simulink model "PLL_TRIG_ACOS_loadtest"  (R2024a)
settings: Solver=VariableStepAuto  StartTime=0.0  StopTime=1  RelTol=1e-3
libraries: spsIGBTDiodeLib x6, spsThreePhaseSeriesRLCBranchLib x6, spsDiodeLib x6, spsGroundLib x4, spsThreePhaseBreakerLib x4, spsThreePhaseVIMeasurementLib x3, spsSeriesRLCBranchLib x3, spsMultimeterLib x3, spsThreePhaseSourceLib x2, spsTHDLib x2, spsPower3phInstantaneousLib x2, spsPVArrayLib x1

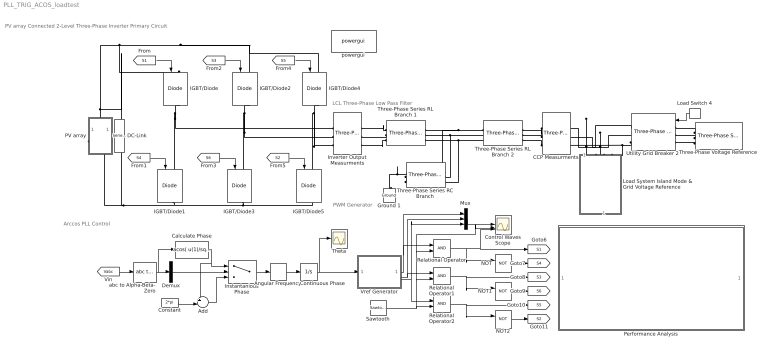
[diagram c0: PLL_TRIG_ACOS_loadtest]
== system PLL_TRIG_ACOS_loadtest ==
  note: PV array Connected 2-Level Three-Phase Inverter Primary Circuit
  note: LCL Three-Phase Low Pass Filter
  note: PWM Generator
  note: Arccos PLL Control
  Add : Sum  Inputs=+-|
  Angular Frequency : Derivative
  CCP Measurments : spsThreePhaseVIMeasurementLib/Three-Phase V-I Measurement  VoltageMeasurement=phase-to-phase  SetLabelV=on  LabelV=Vabc  Vpu=off  VpuLL=off  CurrentMeasurement=yes  SetLabelI=on  LabelI=Iabc  Ipu=off  Pbase=100e6  Vbase=500e3  OutputType=Complex  PhasorSimulation=off  PSBequivalent=0
  Calculate Phase : Fcn  Expr=acos( u(1)/sqrt( u(1)^2 + u(2)^2 ) )
  Constant : Constant  Value=2*pi
  Continuous Phase : Integrator
  Control Waves Scope : Scope  NumInputPorts=3
  DC-Link : spsSeriesRLCBranchLib/Series RLC Branch  LConnTagsString=__new0  RConnTagsString=__new0  BranchType=RC  Resistance=20e-3  Inductance=1e-3  SetiL0=off  InitialCurrent=0  Capacitance=81e-6  Setx0=off  InitialVoltage=0  Measurements=None
  Demux : Demux  Outputs=3
  Ground 1 : spsGroundLib/Ground  LConnTagsString=a
  IGBT/Diode{,1..5} (6 alike) : spsIGBTDiodeLib/IGBT//Diode  Ron=1e-3  Rs=1e5  Cs=inf  Measurements=off
  Instantanious Phase : Switch  Criteria=u2 > Threshold
  Inverter Output Measurments : spsThreePhaseVIMeasurementLib/Three-Phase V-I Measurement  VoltageMeasurement=phase-to-phase  SetLabelV=on  LabelV=Vinv  Vpu=off  VpuLL=off  CurrentMeasurement=yes  SetLabelI=on  LabelI=Iinv  Ipu=off  Pbase=100e6  Vbase=500e3  OutputType=Complex  PhasorSimulation=off  PSBequivalent=0
  Load Switch 4 : DiscretePulseGenerator  PulseType=Time based  Period=1.2  PulseWidth=50  PhaseDelay=0.6
  Load System Island Mode & Grid Voltage Reference : Subsystem
  Mux : Mux  Inputs=3
  NOT : Logic  Operator=NOT  IconShape=distinctive  AllPortsSameDT=off  OutDataTypeStr=boolean
  NOT1 : Logic  Operator=NOT  IconShape=distinctive  AllPortsSameDT=off  OutDataTypeStr=boolean
  NOT2 : Logic  Operator=NOT  IconShape=distinctive  AllPortsSameDT=off  OutDataTypeStr=boolean
  PV array : Subsystem
  Performance Analysis : Subsystem
  Relational Operator : RelationalOperator  OutDataTypeStr=boolean  RndMeth=Simplest
  Relational Operator1 : RelationalOperator  OutDataTypeStr=boolean  RndMeth=Simplest
  Relational Operator2 : RelationalOperator  OutDataTypeStr=boolean  RndMeth=Simplest
  Sawtooth : spsSawtoothGeneratorLib/Sawtooth Generator  Freq=1e4  Phase=0  Ts=0
  Theta : Scope
  Three-Phase Series RC Branch : spsThreePhaseSeriesRLCBranchLib/Three-Phase Series RLC Branch  LConnTagsString=A|B|C  RConnTagsString=A|B|C  BranchType=RC  Resistance=20e-3  Inductance=500e-4  Capacitance=81e-6  Measurements=None
  Three-Phase Series RL Branch 1 : spsThreePhaseSeriesRLCBranchLib/Three-Phase Series RLC Branch  LConnTagsString=A|B|C  RConnTagsString=A|B|C  BranchType=RL  Resistance=20e-3  Inductance=45e-6  Capacitance=1e-6  Measurements=None
  Three-Phase Series RL Branch 2 : spsThreePhaseSeriesRLCBranchLib/Three-Phase Series RLC Branch  LConnTagsString=A|B|C  RConnTagsString=A|B|C  BranchType=RL  Resistance=20e-3  Inductance=45e-6  Capacitance=1e-6  Measurements=None
  Three-Phase Voltage Reference : spsThreePhaseSourceLib/Three-Phase Source  InternalConnection=Yg  VoltagePhases=off  Voltage=240  PhaseAngle=0  Voltage_phases=[25e3 25e3 25e3]/sqrt(3)  PhaseAngles_phases=[0 -120 +120]  Frequency=50  NonIdealSource=on  SpecifyImpedance=off  Resistance=0.8929  Inductance=16.58e-3  ShortCircuitLevel=100e6  BaseVoltage=240  XRratio=7  BusType=swing  Pref=10e3  Qref=0  Prefabc=[10e3, 10e3, 10e3]  Qrefabc=[0, 0, 0]  Qmin=-inf  Qmax=inf
  Utility Grid Breaker 2 : spsThreePhaseBreakerLib/Three-Phase Breaker  InitialState=open  SwitchA=on  SwitchB=on  SwitchC=on  SwitchTimes="[1/60  5/60]"  External=on  BreakerResistance=0.01  SnubberResistance=1e6  SnubberCapacitance=inf  Measurements=None
  Vref Generator : Subsystem
  abc to Alpha-Beta-Zero : spsabctoAlphaBetaZeroLib/abc to Alpha-Beta-Zero
  powergui : spspowerguiLib/powergui  Priority=1  SimulationMode=Discrete  SampleTime=1e-6  frequency=50  Iterations=50  frequencyindice=0  Pbase=100e6  ErrMax=1e-4  UnitsV=kV  UnitsW=MW  buscounter=0  FunctionMessages=off  echomessages=off  EnableUseOfTLC=off  CurrentSourceSwitches=off  DisableSnubberDevices=off  DisableRonSwitches=off  DisableVfSwitches=off  DisplayEquations=off  AutomaticDiscreteSolvers=off  SolverType=Tustin/Backward Euler (TBE)  Interpol=off  ExternalGateDelay=off  methode=off  Ts=100  x0status=blocks  SPID=on  SwTol=0  HookPort=off  NonlinearTolerance=1e-4  nMaxIteration=100  ContinueOnMaxIteration=off  RestoreLinks=warning  ResistiveCurrentMeasurement=off  Frange=[0:2:500]  Ylog=off  Xlog=on  ShowGrid=off  save=off  variable=ZData  structure=0  ZoomFFT=off  StartTime=0.0  cycles=1  DisplayStyle=1  fundamental=60  FreqAxis=off  MaxFrequency=1000  frequencyindicesteady=1  RmsSteady=1  display=off
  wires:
  [Vabc] -> abc to Alpha-Beta-Zero/1
  Load Switch 4/1 -> Utility Grid Breaker 2/1
  Relational Operator/1 -> [S1], Control Waves Scope/3, NOT/1
  NOT2/1 -> [S2]
  Vref Generator/1(Out1) -> Relational Operator/1, Mux/1
  Vref Generator/3(Out3) -> Relational Operator2/1, Mux/3
  NOT1/1 -> [S6]
  Sawtooth/1 -> Relational Operator2/2, Relational Operator1/2, Control Waves Scope/2, Relational Operator/2
  [S5] -> IGBT/Diode4/1
  Vref Generator/2(Out2) -> Relational Operator1/1, Mux/2
  [S4] -> IGBT/Diode1/1
  Relational Operator2/1 -> [S5], NOT2/1
  Relational Operator1/1 -> [S3], NOT1/1
  [S1] -> IGBT/Diode/1
  [S6] -> IGBT/Diode3/1
  Mux/1 -> Control Waves Scope/1
  [S2] -> IGBT/Diode5/1
  [S3] -> IGBT/Diode2/1
  NOT/1 -> [S4]
  abc to Alpha-Beta-Zero/1 -> Calculate Phase/1, Demux/1
  Constant/1 -> Add/2
  Calculate Phase/1 -> Instantanious Phase/1, Add/1
  Add/1 -> Instantanious Phase/3
  Demux/2 -> Instantanious Phase/2
  Instantanious Phase/1 -> Angular Frequency/1
  Continuous Phase/1 -> Theta/1, Vref Generator/1(Input)
  Angular Frequency/1 -> Continuous Phase/1
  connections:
  Utility Grid Breaker 2/RConn3 -- Load System Island Mode & Grid Voltage Reference/LConn3 -- CCP Measurments/RConn3
  IGBT/Diode3/RConn1 -- PV array/RConn1 -- DC-Link/RConn1 -- IGBT/Diode1/RConn1 -- IGBT/Diode5/RConn1
  Three-Phase Series RC Branch/RConn2 -- Ground 1/LConn1 -- Three-Phase Series RC Branch/RConn1 -- Three-Phase Series RC Branch/RConn3
  Three-Phase Series RL Branch 2/LConn1 -- Three-Phase Series RC Branch/LConn1 -- Three-Phase Series RL Branch 1/RConn1
  Three-Phase Series RC Branch/LConn2 -- Three-Phase Series RL Branch 1/RConn2 -- Three-Phase Series RL Branch 2/LConn2
  PV array/LConn1 -- IGBT/Diode/LConn1 -- IGBT/Diode2/LConn1 -- IGBT/Diode4/LConn1 -- DC-Link/LConn1
  Three-Phase Series RC Branch/LConn3 -- Three-Phase Series RL Branch 1/RConn3 -- Three-Phase Series RL Branch 2/LConn3
  IGBT/Diode2/RConn1 -- Inverter Output Measurments/LConn2 -- IGBT/Diode3/LConn1
  Load System Island Mode & Grid Voltage Reference/LConn2 -- CCP Measurments/RConn2 -- Utility Grid Breaker 2/RConn2
  Load System Island Mode & Grid Voltage Reference/LConn1 -- CCP Measurments/RConn1 -- Utility Grid Breaker 2/RConn1
  IGBT/Diode4/RConn1 -- Inverter Output Measurments/LConn3 -- IGBT/Diode5/LConn1
  IGBT/Diode/RConn1 -- Inverter Output Measurments/LConn1 -- IGBT/Diode1/LConn1
  Three-Phase Voltage Reference/RConn3 -- Utility Grid Breaker 2/LConn3
  CCP Measurments/LConn1 -- Three-Phase Series RL Branch 2/RConn1
  Three-Phase Voltage Reference/RConn1 -- Utility Grid Breaker 2/LConn1
  Three-Phase Series RL Branch 1/LConn2 -- Inverter Output Measurments/RConn2
  Three-Phase Series RL Branch 1/LConn3 -- Inverter Output Measurments/RConn3
  CCP Measurments/LConn3 -- Three-Phase Series RL Branch 2/RConn3
  CCP Measurments/LConn2 -- Three-Phase Series RL Branch 2/RConn2
  Three-Phase Voltage Reference/RConn2 -- Utility Grid Breaker 2/LConn2
  Three-Phase Series RL Branch 1/LConn1 -- Inverter Output Measurments/RConn1

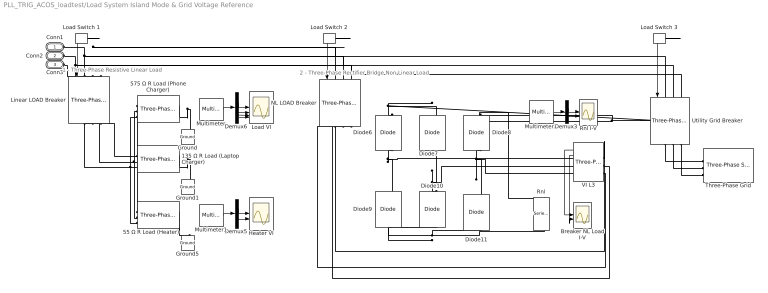
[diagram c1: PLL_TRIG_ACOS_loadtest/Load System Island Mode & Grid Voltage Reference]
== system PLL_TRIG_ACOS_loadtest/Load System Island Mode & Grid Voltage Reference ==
  note: 1 - Three-Phase Resistive Linear Load
  note: 2 - Three-Phase Rectifier Bridge Non-Linear Load
  135 Ω R Load (Laptop Charger) : spsThreePhaseSeriesRLCBranchLib/Three-Phase Series RLC Branch  LConnTagsString=A|B|C  RConnTagsString=A|B|C  BranchType=R  Resistance=135  Inductance=5.1e-3  Capacitance=1e-6  Measurements=Branch voltages and currents
  55 Ω R Load (Heater) : spsThreePhaseSeriesRLCBranchLib/Three-Phase Series RLC Branch  LConnTagsString=A|B|C  RConnTagsString=A|B|C  BranchType=R  Resistance=55  Inductance=5.1e-3  Capacitance=1e-6  Measurements=Branch voltages and currents
  575 Ω R Load (Phone Charger) : spsThreePhaseSeriesRLCBranchLib/Three-Phase Series RLC Branch  LConnTagsString=A|B|C  RConnTagsString=A|B|C  BranchType=R  Resistance=575  Inductance=5.1e-3  Capacitance=1e-6  Measurements=Branch voltages and currents
  Breaker NL Load I-V : Scope  NumInputPorts=2
  Demux3 : Demux  Outputs=2
  Demux5 : Demux  Outputs=2
  Demux6 : Demux
  Diode{6..11} (6 alike) : spsDiodeLib/Diode  Ron=0.001  Lon=0  Vf=0.8  IC=0  UseSnubber=0  Rs=10e+6  Cs=250e-9  Measurements=off
  Ground : spsGroundLib/Ground  LConnTagsString=a
  Ground1 : spsGroundLib/Ground  LConnTagsString=a
  Ground5 : spsGroundLib/Ground  LConnTagsString=a
  Heater VI : Scope  NumInputPorts=2
  Linear LOAD Breaker : spsThreePhaseBreakerLib/Three-Phase Breaker  InitialState=open  SwitchA=on  SwitchB=on  SwitchC=on  SwitchTimes="[1/60  5/60]"  External=on  BreakerResistance=0.01  SnubberResistance=1e6  SnubberCapacitance=inf  Measurements=None
  Load Switch 1 : DiscretePulseGenerator  PulseType=Time based  Period=0.6  PulseWidth=100/3
  Load Switch 2 : DiscretePulseGenerator  PulseType=Time based  Period=0.6  PulseWidth=100/3  PhaseDelay=0.2
  Load Switch 3 : DiscretePulseGenerator  PulseType=Time based  Period=0.6  PulseWidth=100/3  PhaseDelay=0.4
  Load VI : Scope  NumInputPorts=4
  Multimeter : spsMultimeterLib/Multimeter  L=20  sel=[8 2 18 12]  yselected={}  Gain=[1 1 1 1]  OutputType=Complex  PlotAtSimulationStop=off  PhasorSimulation=off
  Multimeter1 : spsMultimeterLib/Multimeter  L=20  sel=[5 15]  yselected={}  Gain=[1 1]  OutputType=Complex  PlotAtSimulationStop=off  PhasorSimulation=off
  Multimeter2 : spsMultimeterLib/Multimeter  L=20  sel=[1 11]  yselected={}  Gain=[1 1]  OutputType=Complex  PlotAtSimulationStop=off  PhasorSimulation=off
  NL LOAD Breaker : spsThreePhaseBreakerLib/Three-Phase Breaker  InitialState=open  SwitchA=on  SwitchB=on  SwitchC=on  SwitchTimes="[1/60  5/60]"  External=on  BreakerResistance=0.01  SnubberResistance=1e6  SnubberCapacitance=inf  Measurements=None
  Rnl : spsSeriesRLCBranchLib/Series RLC Branch  LConnTagsString=__new0  RConnTagsString=__new0  BranchType=R  Resistance=60  Inductance=1e-6  SetiL0=off  InitialCurrent=0  Capacitance=0.01598  Setx0=off  InitialVoltage=0  Measurements=Branch voltage and current
  Rnl I-V : Scope  NumInputPorts=2
  Three-Phase Grid : spsThreePhaseSourceLib/Three-Phase Source  InternalConnection=Yg  VoltagePhases=off  Voltage=240  PhaseAngle=0  Voltage_phases=[25e3 25e3 25e3]/sqrt(3)  PhaseAngles_phases=[0 -120 +120]  Frequency=50  NonIdealSource=on  SpecifyImpedance=off  Resistance=0.8929  Inductance=16.58e-3  ShortCircuitLevel=100e6  BaseVoltage=240  XRratio=7  BusType=swing  Pref=10e3  Qref=0  Prefabc=[10e3, 10e3, 10e3]  Qrefabc=[0, 0, 0]  Qmin=-inf  Qmax=inf
  Utility Grid Breaker : spsThreePhaseBreakerLib/Three-Phase Breaker  InitialState=open  SwitchA=on  SwitchB=on  SwitchC=on  SwitchTimes="[1/60  5/60]"  External=on  BreakerResistance=0.01  SnubberResistance=1e6  SnubberCapacitance=inf  Measurements=None
  VI L3 : spsThreePhaseVIMeasurementLib/Three-Phase V-I Measurement  VoltageMeasurement=phase-to-phase  SetLabelV=off  LabelV=Vabc  Vpu=off  VpuLL=off  CurrentMeasurement=yes  SetLabelI=off  LabelI=Iabc  Ipu=off  Pbase=100e6  Vbase=500e3  OutputType=Complex  PhasorSimulation=off  PSBequivalent=0
  Conn1 : PMIOPort  Side=Left
  Conn2 : PMIOPort  Port=2  Side=Left
  Conn3 : PMIOPort  Port=3  Side=Left
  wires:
  Demux5/2 -> Heater VI/2
  Demux6/2 -> Load VI/2
  Demux6/4 -> Load VI/4
  Demux6/1 -> Load VI/1
  Multimeter/1 -> Demux6/1
  Demux6/3 -> Load VI/3
  Demux5/1 -> Heater VI/1
  Multimeter1/1 -> Demux5/1
  Load Switch 3/1 -> Utility Grid Breaker/1
  Multimeter2/1 -> Demux3/1
  Demux3/1 -> Rnl I-V/1
  Demux3/2 -> Rnl I-V/2
  VI L3/2 -> Breaker NL Load I-V/2
  VI L3/1 -> Breaker NL Load I-V/1
  Load Switch 1/1 -> Linear LOAD Breaker/1
  Load Switch 2/1 -> NL LOAD Breaker/1
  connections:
  55 Ω R Load (Heater)/LConn2 -- 135 Ω R Load (Laptop Charger)/LConn2 -- Linear LOAD Breaker/RConn2 -- 575 Ω R Load (Phone Charger)/LConn2
  55 Ω R Load (Heater)/LConn3 -- 135 Ω R Load (Laptop Charger)/LConn3 -- Linear LOAD Breaker/RConn3 -- 575 Ω R Load (Phone Charger)/LConn3
  55 Ω R Load (Heater)/RConn1 -- 55 Ω R Load (Heater)/RConn2 -- 55 Ω R Load (Heater)/RConn3 -- Ground5/LConn1
  55 Ω R Load (Heater)/LConn1 -- 135 Ω R Load (Laptop Charger)/LConn1 -- Linear LOAD Breaker/RConn1 -- 575 Ω R Load (Phone Charger)/LConn1
  575 Ω R Load (Phone Charger)/RConn1 -- Ground/LConn1 -- 575 Ω R Load (Phone Charger)/RConn3 -- 575 Ω R Load (Phone Charger)/RConn2
  135 Ω R Load (Laptop Charger)/RConn1 -- Ground1/LConn1 -- 135 Ω R Load (Laptop Charger)/RConn3 -- 135 Ω R Load (Laptop Charger)/RConn2
  Utility Grid Breaker/RConn1 -- Three-Phase Grid/RConn1
  Utility Grid Breaker/RConn3 -- Three-Phase Grid/RConn3
  Utility Grid Breaker/RConn2 -- Three-Phase Grid/RConn2
  Conn1/RConn1 -- NL LOAD Breaker/LConn1 -- Utility Grid Breaker/LConn1 -- Linear LOAD Breaker/LConn1
  Conn2/RConn1 -- NL LOAD Breaker/LConn2 -- Utility Grid Breaker/LConn2 -- Linear LOAD Breaker/LConn2
  Conn3/RConn1 -- NL LOAD Breaker/LConn3 -- Utility Grid Breaker/LConn3 -- Linear LOAD Breaker/LConn3
  Diode6/RConn1 -- Rnl/LConn1 -- Diode8/RConn1 -- Diode7/RConn1
  Diode6/LConn1 -- Diode9/RConn1 -- VI L3/RConn1
  Diode8/LConn1 -- Diode11/RConn1 -- VI L3/RConn3
  Diode9/LConn1 -- Rnl/RConn1 -- Diode11/LConn1 -- Diode10/LConn1
  Diode10/RConn1 -- Diode7/LConn1 -- VI L3/RConn2
  NL LOAD Breaker/RConn1 -- VI L3/LConn1
  VI L3/LConn2 -- NL LOAD Breaker/RConn2
  VI L3/LConn3 -- NL LOAD Breaker/RConn3

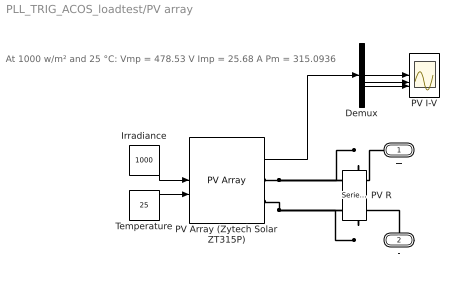
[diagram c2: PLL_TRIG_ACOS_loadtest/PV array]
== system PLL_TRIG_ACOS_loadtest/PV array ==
  note: At 1000 w/m² and 25 °C: Vmp = 478.53 V Imp = 25.68 A Pm = 315.0936
  Demux : Demux  Outputs=5
  Irradiance : Constant  Value=1000
  PV I-V : Scope  NumInputPorts=5
  PV Array (Zytech Solar ZT315P) : spsPVArrayLib/PV Array  Npar=3  Nser=13  PlotType=array @ 25 deg.C & specified irradiances  S_vec="[ 1000  500  100 ]"  Temp_C_vec="[ 45 25  ]"  ModuleName=Zytech Solar ZT315P  PlotWhenSelected=off  Pm=315.0936  Ncell=72  Voc=46.44  Isc=9.01  Vm=36.81  Im=8.56  beta_Voc_pc=-0.3199  alpha_Isc_pc=0.048302  beta_Voc=-0.14856  alpha_Isc=0.004352  IL=9.0792  I0=6.901e-11  nI=0.9809  Rsh=572.7811  Rs=0.50125  RobustModel=off  RobustCellTemperature=313.3991  BAL=on  Tc=1e-6  Tfilter=5e-5
  PV R : spsSeriesRLCBranchLib/Series RLC Branch  LConnTagsString=__new0  RConnTagsString=__new0  BranchType=R  Resistance=18.6  Inductance=1e-3  SetiL0=off  InitialCurrent=0  Capacitance=1e-6  Setx0=off  InitialVoltage=0  Measurements=None
  Temperature : Constant  Value=25
  + : PMIOPort  Side=Left
  - : PMIOPort  Port=2  Side=Right
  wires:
  PV Array (Zytech Solar ZT315P)/1 -> Demux/1
  Demux/3 -> PV I-V/3
  Temperature/1 -> PV Array (Zytech Solar ZT315P)/2
  Demux/2 -> PV I-V/2
  Irradiance/1 -> PV Array (Zytech Solar ZT315P)/1
  Demux/1 -> PV I-V/1
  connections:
  PV Array (Zytech Solar ZT315P)/RConn1 -- PV R/LConn1 -- +/RConn1
  PV Array (Zytech Solar ZT315P)/RConn2 -- PV R/RConn1 -- -/RConn1

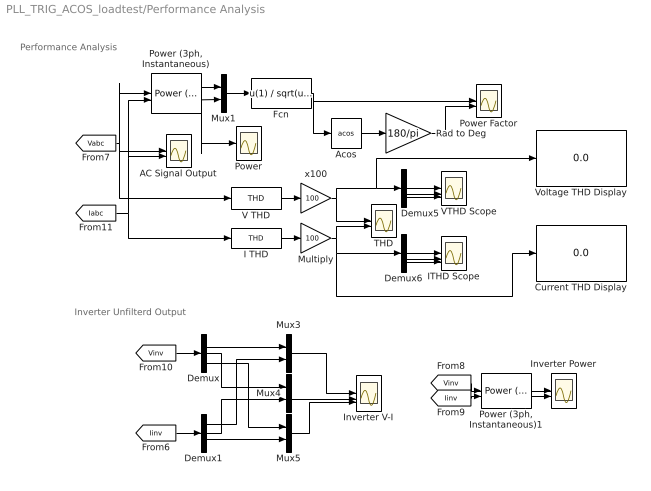
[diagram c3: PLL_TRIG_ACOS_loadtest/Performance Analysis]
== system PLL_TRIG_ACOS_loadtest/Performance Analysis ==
  note: Inverter Unfilterd Output
  note: Performance Analysis
  AC Signal Output : Scope  NumInputPorts=2
  Acos : Trigonometry  Operator=acos
  Current THD Display : Display
  Demux{,1,5..6} (4 alike) : Demux  Outputs=3
  Fcn : Fcn  Expr=u(1) / sqrt(u(1)^2 + u(2)^2)
  I THD : spsTHDLib/THD  Freq=50  Ts=0
  ITHD Scope : Scope  NumInputPorts=3
  Inverter V-I : Scope  NumInputPorts=3
  Inverter Power : Scope  NumInputPorts=2
  Multiply : Gain  Gain=100
  Mux{1,3..5} (4 alike) : Mux  Inputs=2
  Power : Scope
  "Power (3ph, Instantaneous)" : spsPower3phInstantaneousLib/Power (3ph, Instantaneous)
  "Power (3ph, Instantaneous)1" : spsPower3phInstantaneousLib/Power (3ph, Instantaneous)
  Power Factor : Scope  NumInputPorts=2
  Rad to Deg : Gain  Gain=180/pi
  THD : Scope  NumInputPorts=2
  V THD : spsTHDLib/THD  Freq=50  Ts=0
  VTHD Scope : Scope  NumInputPorts=3
  Voltage THD Display : Display
  x100 : Gain  Gain=100
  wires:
  x100/1 -> THD/1, Voltage THD Display/1, Demux5/1
  Fcn/1 -> Power Factor/1, Acos/1
  Demux5/2 -> VTHD Scope/2
  [Iabc] -> I THD/1, "Power (3ph, Instantaneous)"/2, AC Signal Output/2
  Demux6/3 -> ITHD Scope/3
  "Power (3ph, Instantaneous)"/1 -> Power/1, Mux1/1
  Demux6/2 -> ITHD Scope/2
  Multiply/1 -> Current THD Display/1, Demux6/1, THD/2
  Demux5/1 -> VTHD Scope/1
  Rad to Deg/1 -> Power Factor/2
  V THD/1 -> x100/1
  I THD/1 -> Multiply/1
  Demux5/3 -> VTHD Scope/3
  [Vabc] -> V THD/1, AC Signal Output/1, "Power (3ph, Instantaneous)"/1
  "Power (3ph, Instantaneous)"/2 -> Mux1/2
  Acos/1 -> Rad to Deg/1
  Mux1/1 -> Fcn/1
  Demux6/1 -> ITHD Scope/1
  "Power (3ph, Instantaneous)1"/1 -> Inverter Power/1
  "Power (3ph, Instantaneous)1"/2 -> Inverter Power/2
  [Iinv] -> "Power (3ph, Instantaneous)1"/2
  [Vinv] -> "Power (3ph, Instantaneous)1"/1
  Mux3/1 -> Inverter V-I/1
  Mux4/1 -> Inverter V-I/2
  Demux1/3 -> Mux5/2
  Demux1/1 -> Mux3/2
  [Vinv] -> Demux/1
  Demux/3 -> Mux5/1
  Demux/1 -> Mux3/1
  Demux1/2 -> Mux4/2
  Demux/2 -> Mux4/1
  Mux5/1 -> Inverter V-I/3
  [Iinv] -> Demux1/1

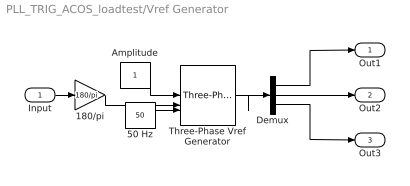
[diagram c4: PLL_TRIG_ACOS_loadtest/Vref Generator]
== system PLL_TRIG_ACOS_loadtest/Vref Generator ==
  Input : Inport
  180/pi : Gain  Gain=180/pi
  50 Hz : Constant  Value=50  VectorParams1D=off  SampleTime=-1
  Amplitude : Constant  VectorParams1D=off  SampleTime=-1
  Demux : Demux  Outputs=3
  Three-Phase Vref Generator : spsThreePhaseSineGeneratorLib/Three-Phase Sine Generator  Ts=0
  Out1 : Outport
  Out2 : Outport  Port=2
  Out3 : Outport  Port=3
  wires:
  Amplitude/1 -> Three-Phase Vref Generator/1
  Three-Phase Vref Generator/1 -> Demux/1
  Demux/1 -> Out1/1
  Demux/2 -> Out2/1
  Demux/3 -> Out3/1
  50 Hz/1 -> Three-Phase Vref Generator/3
  Input/1 -> 180/pi/1
  180/pi/1 -> Three-Phase Vref Generator/2
